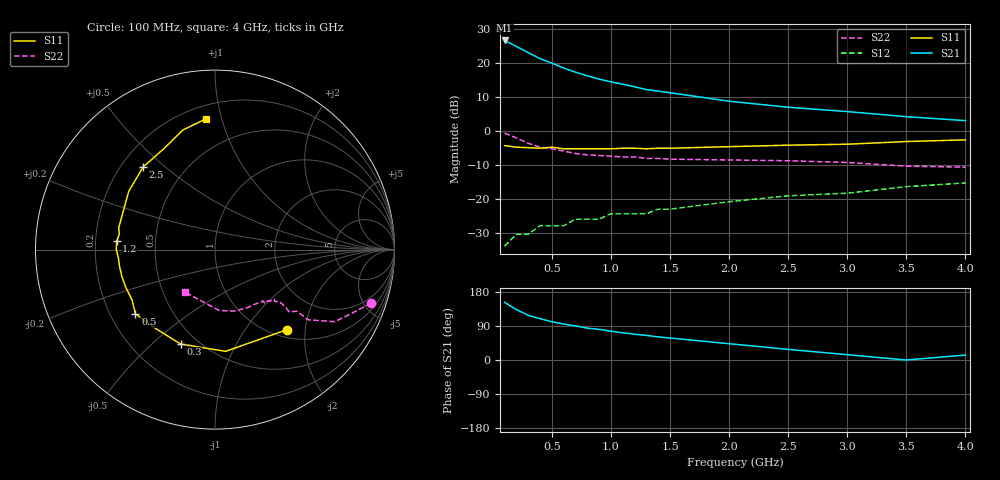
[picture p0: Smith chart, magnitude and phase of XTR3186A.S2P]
! HXTR-3186
! Typical S-Parameters  Vce =10 V, Ic = 10 mA
# ghz s ma r 50
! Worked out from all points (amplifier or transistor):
!   20 points, 100 MHz to 4 GHz, reference 50 ohm
!   highest |S21| = 26.5 dB at 100 MHz (marker M1)
!   |S21| within 3 dB of that: start of sweep to 268.5 MHz
!   unconditionally stable (mu >= 1): 1.183 GHz to 3.269 GHz
!   at 400 MHz: K = 0.51, MSG = 24.5 dB, |S12| = -28.0 dB
!   at 1.1 GHz: K = 0.94, MSG = 19.0 dB, |S12| = -24.4 dB
!   at 4 GHz: K = 0.95, MSG = 9.2 dB, |S12| = -15.4 dB
!   S11 on the Smith chart (normalised r, x): 100 MHz: 1.15, -1.60; 300 MHz: 0.40, -0.62; 500 MHz: 0.31, -0.32; 1.2 GHz: 0.29, +0.04; 2.5 GHz: 0.29, +0.42; 4 GHz: 0.29, +0.89
0.1  0.6 -48.0  21.1 152.0  0.02 69.0  0.92 -19.0
0.2  0.57 -84.0  17.2 133.0  0.03 56.0  0.78 -31.0
0.3  0.56 -110.0  14 118.0  0.03 48.0  0.65 -37.0
0.4  0.55 -127.0  11.4 109.0  0.04 45.0  0.57 -37.0
0.5  0.57 -141.0  9.8 101.0  0.04 43.0  0.54 -40.0
0.6  0.54 -149.0  8.3 95.0  0.04 44.0  0.5 -39.0
0.7  0.54 -157.0  7.2 90.0  0.05 43.0  0.46 -39.0
0.8  0.54 -164.0  6.4 84.0  0.05 44.0  0.44 -41.0
0.9  0.54 -170.0  5.7 81.0  0.05 44.0  0.43 -40.0
1  0.54 -175.0  5.2 76.0  0.06 45.0  0.42 -43.0
1.1  0.55 180.0  4.8 72.0  0.06 45.0  0.41 -44.0
1.2  0.55 175.0  4.4 68.0  0.06 45.0  0.41 -47.0
1.3  0.54 171.0  4 65.0  0.06 46.0  0.39 -47.0
1.4  0.55 167.0  3.8 61.0  0.07 46.0  0.39 -49.0
1.5  0.55 162.0  3.6 58.0  0.07 46.0  0.38 -52.0
2  0.58 146.0  2.7 43.0  0.09 45.0  0.37 -61.0
2.5  0.61 131.0  2.2 28.0  0.11 43.0  0.36 -72.0
3  0.63 117.0  1.9 14.0  0.12 39.0  0.34 -86.0
3.5  0.69 105.0  1.6 0.0  0.15 34.0  0.3 -102.0
4  0.73 94.0  1.4 13.0  0.17 28.0  0.29 -125.0
